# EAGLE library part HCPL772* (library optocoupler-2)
40 ns Propagation Delay, CMOS Optocoupler *Pin 3 is the anode of the internal LED and must be left unconnected for guaranteed data sheet perfomance. Pin 7 is not connected internally. Source: HCPL7721.pdf
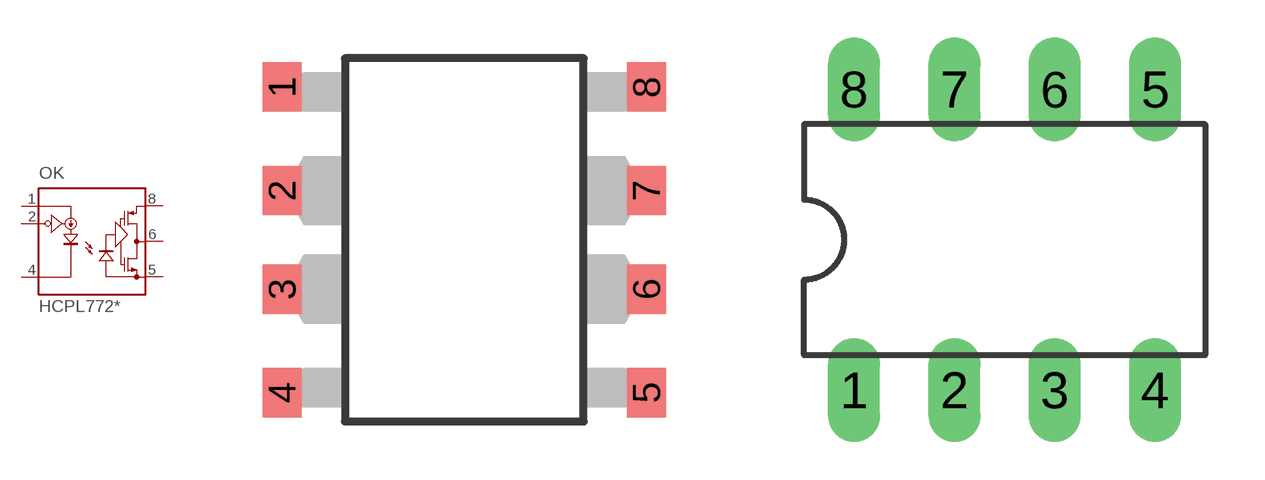
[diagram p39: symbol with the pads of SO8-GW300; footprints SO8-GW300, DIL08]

Designator prefix OK

## HCPL7720#300, HCPL7721#300  [SO8-GW300]
1  VDD1  pas
2  VI  in
4  GND1  pas
5  GND2  pas
6  VO  pas
8  VDD2  pas

## HCPL7720, HCPL7721  [DIL08]
Pads as for SO8-GW300

## HCPL7720SO8, HCPL7721SO8  [SO-8]
Pads as for SO8-GW300

## Footprint SO8-GW300 (pad centres in mm)
HCPL-772X Package witch Gull Wing Surface Mount Option 300 Source: HCPL7221.pdf
smd 1 x 1.27: 1 -4.69,3.937; 2 -4.69,1.27; 3 -4.69,-1.27; 4 -4.69,-3.937; 5 4.69,-3.937; 6 4.69,-1.27; 7 4.69,1.27; 8 4.69,3.937

## Footprint DIL08 (pad centres in mm)
Dual In Line Package
drill 0.813 long: 1 -3.81,-3.81; 2 -1.27,-3.81; 3 1.27,-3.81; 4 3.81,-3.81; 5 3.81,3.81; 6 1.27,3.81; 7 -1.27,3.81; 8 -3.81,3.81

## Footprint SO-8 (pad centres in mm)
Small Outline SO-8 Packages Source: HCPL7221.pdf
smd 0.7 x 0.45: 1 -2.79,1.905; 2 -2.79,0.635; 3 -2.79,-0.635; 4 -2.79,-1.905; 5 2.79,-1.905; 6 2.79,-0.635; 7 2.79,0.635; 8 2.79,1.905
